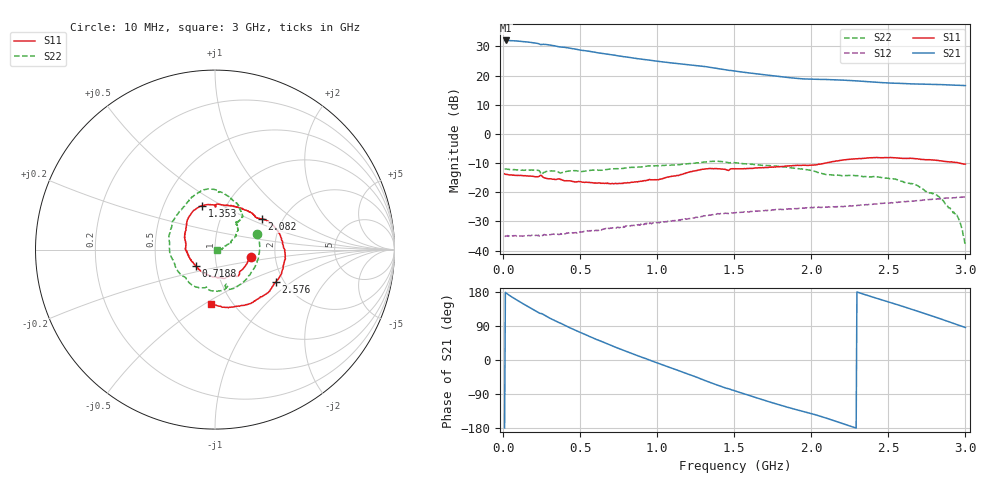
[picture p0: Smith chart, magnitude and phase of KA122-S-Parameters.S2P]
!Agilent Technologies,E5071B,JP1KK00126,A.08.11
!Date: Thu Jun 15 20:16:37 2023
!Data & Calibration Information:
!Freq	S11:SOLT2(ON)	S21:SOLT2(ON)	S12:SOLT2(ON)	S22:SOLT2(ON)
# Hz S dB R 50
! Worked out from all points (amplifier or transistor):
!   600 points, 10 MHz to 3 GHz, reference 50 ohm
!   highest |S21| = 32.1 dB at 19.98 MHz (marker M1)
!   |S21| within 3 dB of that: start of sweep to 471.9 MHz
!   unconditionally stable (mu >= 1): start of sweep to 1.183 GHz; 1.587 GHz to 1.606 GHz; 1.609 GHz to end of sweep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
!   at 509.2 MHz: K = 1.09, MAG = 29.3 dB, |S12| = -33.6 dB
!   at 1.507 GHz: K = 0.97, MSG = 24.3 dB, |S12| = -27.0 dB
!   at 3 GHz: K = 1.09, MAG = 17.3 dB, |S12| = -21.6 dB
!   S11 on the Smith chart (normalised r, x): 10 MHz: 1.50, -0.13; 718.8 MHz: 0.80, -0.15; 1.353 GHz: 0.77, +0.40; 2.082 GHz: 1.57, +0.59; 2.576 GHz: 1.82, -0.77; 3 GHz: 0.80, -0.53
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1e7  -13.69 -11.9  32.04 -179.2  -35.20 4.8  -11.99 20.7
1.998331e7  -13.85 -9.6  32.06 176.7  -35.04 2.1  -12.05 6.2
1.148247e8  -14.22 -23.7  31.75 152.0  -34.97 -4.0  -12.44 -31.8
1.697329e8  -14.44 -33.4  31.46 139.1  -34.83 -5.8  -12.38 -48.5
2.196494e8  -14.68 -41.5  31.09 127.5  -34.81 -8.2  -12.41 -64.0
3.394491e8  -15.61 -65.3  30.17 102.9  -34.46 -12.4  -12.74 -94.5
4.193155e8  -16.10 -82.6  29.54 87.7  -34.03 -16.5  -12.78 -112.2
5.091653e8  -16.48 -98.3  28.69 71.4  -33.60 -20.5  -12.91 -136.2
5.940234e8  -16.90 -112.9  28.03 56.2  -33.17 -26.0  -12.42 -153.9
7.188147e8  -17.04 -138.7  27.03 35.5  -32.18 -33.1  -11.93 -177.3
8.43606e8  -16.56 -161.6  26.05 16.0  -31.38 -41.9  -11.44 161.7
1.008331e9  -15.71 169.0  24.89 -8.9  -30.38 -54.7  -10.89 138.6
1.193022e9  -13.32 136.7  23.79 -36.2  -29.22 -70.2  -10.24 118.8
1.352755e9  -11.87 106.5  22.77 -60.7  -27.70 -85.8  -9.40 101.4
1.507496e9  -11.92 83.5  21.54 -82.0  -27.02 -104.5  -9.88 83.2
1.73212e9  -11.41 60.7  20.07 -110.9  -26.13 -128.6  -10.86 65.4
2.006661e9  -10.68 37.3  18.76 -142.2  -25.29 -157.6  -12.61 50.1
2.081536e9  -10.13 33.2  18.68 -151.3  -25.07 -167.2  -13.78 50.3
2.291185e9  -8.50 9.5  18.21 -179.7  -24.61 173.5  -14.32 51.8
2.505826e9  -8.13 -18.8  17.47 152.6  -23.70 150.4  -15.30 42.3
2.57571e9  -8.31 -27.8  17.34 143.7  -23.32 143.4  -16.01 38.9
3e9  -10.34 -94.5  16.58 85.6  -21.61 92.9  -38.48 -21.2
